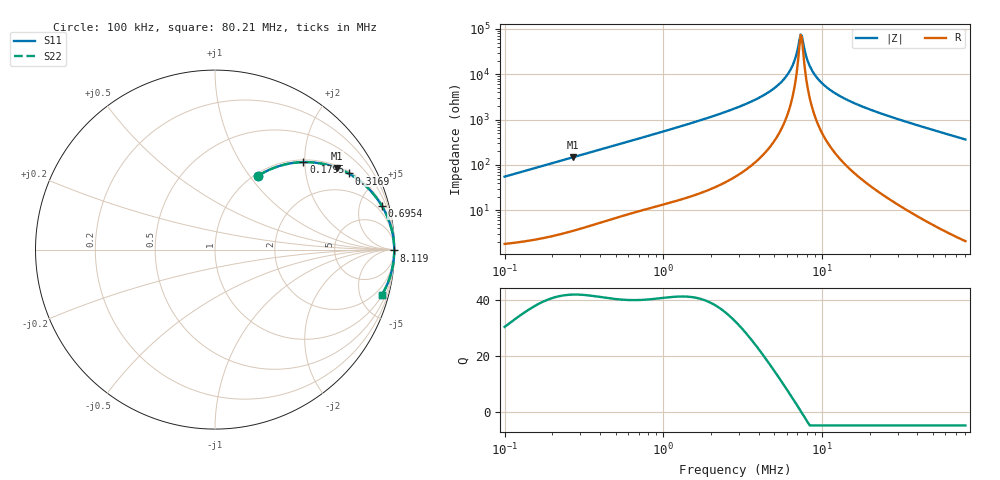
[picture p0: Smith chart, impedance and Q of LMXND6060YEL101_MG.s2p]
! LMXND6060YEL101_MG  S-PARAMETER MODEL  ( General Type )
! Model Generated by TAIYO YUDEN Corporation (https://www.yuden.co.jp/en/)
! Version 1.0
! TAIYO YUDEN Control No. 191025NI43SB-FBB
! Copyright(c) 2019 TAIYO YUDEN CO.,LTD. All Rights Reserved.
! Product Description (link to TY-COMPAS)
! https://ds.yuden.co.jp/TYCOMPAS/or/detail?pn=LMXND6060YEL101MMG&u=M
! Products Name : Inductors
! Characteristics :
!  Inductance : 100 uH , SRF(min) : 3.0 MHz , DC Resistance(max) : 0.6058 Ohm
!  Rated Current : Saturation :900 mA , Temp Rise : 750 mA (40 degC)
!  Case Size : 6.0 x 6.0 / 0.236 x 0.236 [mm/inch] , Thickness : 4.5 / 0.177 [mm/inch]
!  (Conditions: Temperature = 25 degC , DC Bias Current/Voltage = 0A / 0V)
! External Node Assignments :
!  1  o---GGG---o  2
! GND o---------o GND
! Frequency Range : 0.1MHz  -  80.209071MHz  [ 402 STEP ]
# MHz S RI R 50
! Freq[MHz].  S11 Real  S11 Imag  S21 Real  S21 Imag  S12 Real  S12 Imag  S22 Real  S22 Imag
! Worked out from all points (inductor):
!   401 points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, 100 kHz to 80.21 MHz, reference 50 ohm
!   read as one part in series: L = 87.4 uH near 103.4 kHz
!   highest Q = 42 at 268.1 kHz (marker M1), where L = 87.1 uH
!   self-resonance near 7.345 MHz
!   S11 on the Smith chart (normalised r, x): 100 kHz: 1.04, +1.10; 179.5 kHz: 1.05, +1.97; 316.9 kHz: 1.08, +3.46; 695.4 kHz: 1.19, +7.57; 8.119 MHz: open; 80.21 MHz: 1.04, -7.29
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0.1  0.2401 0.411  0.7599 -0.411  0.7599 -0.411  0.2401 0.411
0.179523  0.4927 0.4875  0.5073 -0.4875  0.5073 -0.4875  0.4927 0.4875
0.268147  0.679 0.4551  0.321 -0.4551  0.321 -0.4551  0.679 0.4551
0.306519  0.7326 0.4308  0.2674 -0.4308  0.2674 -0.4308  0.7326 0.4308
0.316941  0.7451 0.424  0.2549 -0.424  0.2549 -0.424  0.7451 0.424
0.695384  0.9295 0.2439  0.0705 -0.2439  0.0705 -0.2439  0.9295 0.2439
0.939539  0.9591 0.1861  0.0409 -0.1861  0.0409 -0.1861  0.9591 0.1861
2.832121  0.9951 0.0562  0.00491 -0.0562  0.00491 -0.0562  0.9951 0.0562
4.301557  0.9977 0.0288  0.00228 -0.0288  0.00228 -0.0288  0.9977 0.0288
5.620755  0.9985 0.014  0.00155 -0.014  0.00155 -0.014  0.9985 0.014
6.533406  0.9986 0.00624  0.00136 -0.00624  0.00136 -0.00624  0.9986 0.00624
6.86944  0.9987 0.00368  0.00132 -0.00368  0.00132 -0.00368  0.9987 0.00368
7.222757  0.9987 0.00113  0.0013 -0.00113  0.0013 -0.00113  0.9987 0.00113
7.344523  0.9987 0.000277  0.0013 -0.000277  0.0013 -0.000277  0.9987 0.000277
7.594247  0.9987 -0.00142  0.00129 0.00142  0.00129 0.00142  0.9987 -0.00142
8.119456  0.9987 -0.00483  0.00131 0.00483  0.00131 0.00483  0.9987 -0.00483
8.680988  0.9987 -0.00825  0.00134 0.00825  0.00134 0.00825  0.9987 -0.00825
10.09053  0.9985 -0.0161  0.00152 0.0161  0.00152 0.0161  0.9985 -0.0161
12.54011  0.998 -0.0282  0.00204 0.0282  0.00204 0.0282  0.998 -0.0282
17.22868  0.9964 -0.0483  0.00358 0.0483  0.00358 0.0483  0.9964 -0.0483
26.60888  0.9916 -0.0839  0.00836 0.0839  0.00836 0.0839  0.9916 -0.0839
80.20907  0.9288 -0.2544  0.0712 0.2544  0.0712 0.2544  0.9288 -0.2544
